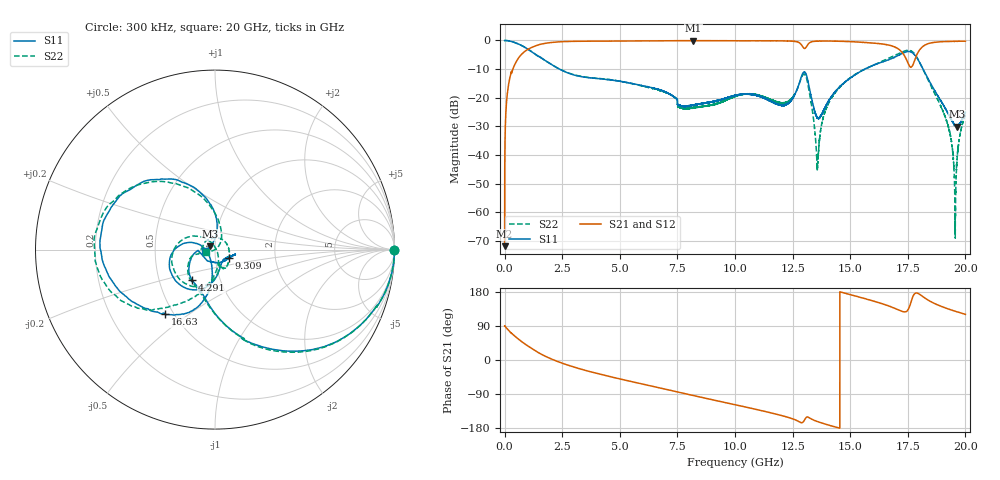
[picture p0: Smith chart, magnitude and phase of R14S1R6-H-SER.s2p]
!{R14S1R6}
!Johanson Technology Inc.
!www.johansontechnology.com
!Test Board Conditions:
!Substrate Type  RO4350B
!Substrate Thickness  20 mil
!Substrate Dk  3.66
!TL Type: GCPW
!TL Trace Width  36 mil
!TL Gap  12 mil
!Electrode orientation  Horizontal
!DUT TOPOLOGY	SERIES
!Mounting Pad LxW  26x36 mil
! Created Wed Nov 25 17:33:21 2020
! 2 Port Network Data from SP1.SP block
! freq  magS11  angS11  magS21  angS21  magS12  angS12  magS22  angS22
# khz S ma R 50
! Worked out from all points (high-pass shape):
!   20001 points, 300 kHz to 20 GHz, reference 50 ohm
!   highest |S21| = -0.06 dB at 8.189 GHz (marker M1); lowest = -71.8 dB at 300 kHz (marker M2)
!   |S21| within 3 dB of the highest: 1.021 GHz to 17.11 GHz (16.09 GHz wide, 177 % of centre); 18.03 GHz to end of sweep
!   lowest |S11| = -30.1 dB at 19.66 GHz (marker M3), VSWR 1.06, Z = 47.4 + j1.66 ohm
!   |S11| at or under -10 dB: 2.384 GHz to 15.63 GHz (13.25 GHz wide, 147 % of centre); 18.16 GHz to end of sweep
!   |S22| runs from -69.0 to 0.0 dB; largest |S21 - S12| = 0.016
!   S11 on the Smith chart (normalised r, x): 300 kHz: open; 4.291 GHz: 0.73, -0.26; 9.309 GHz: 1.16, -0.11; 16.63 GHz: 0.45, -0.41; 20 GHz: 0.90, -0.02
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300  0.9962 -0.3  0.0002573 90.3  0.0003656 95.5  0.9983 -0.1
132300  0.9909 -8.9  0.1319 81.1  0.1326 81.0  0.9906 -8.8
500300  0.9013 -29.3  0.4226 60.0  0.4235 60.1  0.902 -29.4
1717300  0.4588 -78.4  0.8844 11.4  0.8856 11.4  0.4597 -78.5
3334300  0.2335 -112.8  0.969 -24.5  0.9683 -24.5  0.2359 -115.5
4291300  0.2114 -127.4  0.9741 -39.7  0.9734 -39.7  0.2141 -131.3
6667300  0.1407 -160.8  0.9851 -72.8  0.9855 -72.8  0.1373 -163.4
8189300  0.07496 -77.5  0.9933 -93.7  0.9909 -93.6  0.06711 72.2
9309300  0.09119 -31.6  0.9902 -108.8  0.9907 -108.8  0.08105 -9.4
1.00003e7  0.1103 -15.3  0.988 -118.0  0.987 -118.0  0.1049 -45.5
1.21783e7  0.07538 -52.7  0.9798 -149.2  0.9843 -149.0  0.08229 -74.0
1.29963e7  0.2794 -140.5  0.7307 -160.7  0.7338 -160.7  0.2575 -146.8
1.33343e7  0.09305 162.4  0.9485 -156.3  0.9477 -156.2  0.06842 126.9
1.35923e7  0.04416 -157.6  0.9733 -162.7  0.9762 -162.7  0.007683 2.7
1.43423e7  0.1271 -96.8  0.9718 -176.5  0.9758 -176.5  0.1216 -87.2
1.66283e7  0.454 -127.9  0.8377 143.7  0.8271 143.3  0.4809 -135.8
1.66673e7  0.457 -129.1  0.8328 142.7  0.8199 142.5  0.4914 -136.6
1.78443e7  0.5329 133.4  0.5061 176.7  0.5042 177.3  0.5464 137.8
1.91843e7  0.05952 91.5  0.958 136.2  0.9571 136.4  0.03942 47.7
1.95333e7  0.03317 124.3  0.9625 129.2  0.9622 129.2  0.002641 37.0
1.96573e7  0.03126 146.0  0.9657 126.8  0.9645 126.9  0.01041 -154.9
2e7  0.05579 -170.3  0.9701 120.5  0.9676 120.6  0.05073 -162.7
